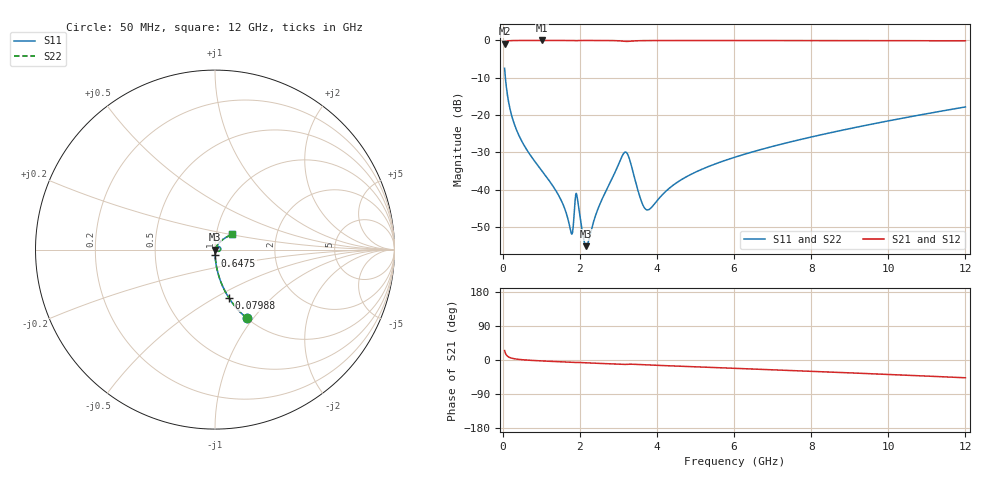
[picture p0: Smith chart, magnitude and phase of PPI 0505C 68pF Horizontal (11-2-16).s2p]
# MHz S MA R 50
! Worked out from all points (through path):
!   1601 points, 50 MHz to 12 GHz, reference 50 ohm
!   highest |S21| = -0.01 dB at 1.013 GHz (marker M1); lowest = -0.9 dB at 50 MHz (marker M2)
!   group delay of S21, straight-line fit = 11.3 ps
!   lowest |S11| = -55.2 dB at 2.164 GHz (marker M3), VSWR 1.00, Z = 50.2 - j0.02 ohm
!   |S11| at or under -10 dB: 69.94 MHz to end of sweep
!   |S22| runs from -55.2 to -7.5 dB; largest |S21 - S12| = 0
!   S11 on the Smith chart (normalised r, x): 50 MHz: 1.00, -0.93; 79.88 MHz: 1.00, -0.58; 647.5 MHz: 1.00, -0.07; 12 GHz: 1.19, +0.21
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50  0.4224 -65.1  0.9061 24.8  0.9061 24.8  0.4224 -65.1
79.875  0.2798 -74.0  0.9597 16.0  0.9597 16.0  0.2798 -74.0
169.5  0.1355 -82.6  0.9903 7.2  0.9903 7.2  0.1355 -82.6
274.0625  0.08345 -85.8  0.996 3.8  0.996 3.8  0.08345 -85.8
647.5  0.03284 -89.0  0.9987 -0.3  0.9987 -0.3  0.03284 -89.0
1013.469  0.01795 -89.5  0.9988 -2.5  0.9988 -2.5  0.01795 -89.5
1498.938  0.007512 -85.7  0.9987 -4.7  0.9987 -4.7  0.007512 -85.7
1767.812  0.002727 -52.2  0.998 -6.0  0.998 -6.0  0.002727 -52.2
1894.781  0.008556 -16.8  0.9915 -6.4  0.9915 -6.4  0.008556 -16.8
1932.125  0.007933 -47.5  0.9939 -6.3  0.9939 -6.3  0.007933 -47.5
2044.156  0.003176 -55.8  0.9978 -6.9  0.9978 -6.9  0.003176 -55.8
2163.656  0.001747 -6.6  0.9981 -7.4  0.9981 -7.4  0.001747 -6.6
2522.156  0.006414 61.2  0.9976 -9.0  0.9976 -9.0  0.006414 61.2
3157  0.03141 19.7  0.9729 -11.8  0.9729 -11.8  0.03141 19.7
3276.5  0.02678 -16.2  0.9731 -11.1  0.9731 -11.1  0.02678 -16.2
3679.812  0.005667 -5.4  0.9941 -12.6  0.9941 -12.6  0.005667 -5.4
4038.312  0.007463 47.9  0.9962 -14.2  0.9962 -14.2  0.007463 47.9
4770.25  0.01493 62.6  0.9969 -17.1  0.9969 -17.1  0.01493 62.6
6025  0.02726 62.5  0.9967 -22.0  0.9967 -22.0  0.02726 62.5
8019.156  0.051 56.8  0.9953 -29.9  0.9953 -29.9  0.051 56.8
10013.31  0.08369 49.6  0.9926 -38.2  0.9926 -38.2  0.08369 49.6
12000  0.1284 41.4  0.9871 -46.9  0.9871 -46.9  0.1284 41.4
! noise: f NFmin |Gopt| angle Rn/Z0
50  0.0003793  0.8613  0.4706  0.000586
1372  0.003935  0.6707  4.76  0.002295
2701  0.009097  0.7133  9.23  0.006218
4031  0.01198  0.6826  13.75  0.00721
5360  0.01194  0.5999  18.09  0.005368
6682  0.01358  0.5728  22.31  0.005558
8012  0.01547  0.5587  26.46  0.005986
9341  0.01745  0.5514  30.49  0.006508
1.067e+04  0.01952  0.5488  34.39  0.007099
1.2e+04  0.02171  0.5499  38.17  0.007764
